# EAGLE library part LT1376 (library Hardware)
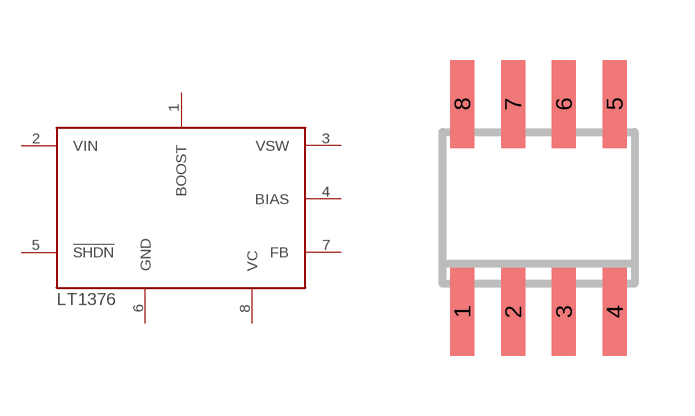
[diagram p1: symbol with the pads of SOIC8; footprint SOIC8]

Designator prefix -

## LT1376  [SOIC8]
1  BOOST
2  VIN
3  VSW
4  BIAS
5  !SHDN
6  GND
7  FB
8  VC

## Footprint SOIC8 (pad centres in mm)
Small Outline IC
smd 0.6 x 2.2: 1 -1.905,-2.6; 2 -0.635,-2.6; 3 0.635,-2.6; 4 1.905,-2.6; 5 1.905,2.6; 6 0.635,2.6; 7 -0.635,2.6; 8 -1.905,2.6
